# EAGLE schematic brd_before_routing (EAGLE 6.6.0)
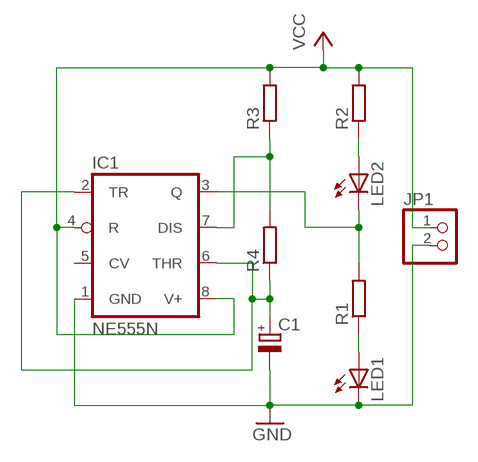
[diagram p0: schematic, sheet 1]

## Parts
C1  CPOL-EUE2.5-6  [E2,5-6]
IC1  NE555N  [DIL08]
JP1  PINHD-1X2  [1X02]
LED1  LED5MM  [LED5MM]
LED2  LED5MM  [LED5MM]
R1  R-EU_0207/10  [0207/10]
R2  R-EU_0207/10  [0207/10]
R3  R-EU_0207/10  [0207/10]
R4  R-EU_0207/10  [0207/10]

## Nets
GND: C1.- IC1.1(GND) JP1.2 LED1.K(C)
N$1: LED2.A R2.1
N$2: IC1.3(Q) LED2.K(C) R1.2
N$3: IC1.7(DIS) R3.1 R4.2
N$4: C1.+ IC1.2(TR) IC1.6(THR) R4.1
N$5: LED1.A R1.1
VCC: IC1.4(R) IC1.8(V+) JP1.1 R2.2 R3.2
Unconnected: IC1.5(CV)

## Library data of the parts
C1 = rcl:CPOL-EU: POLARIZED CAPACITOR, European symbol
IC1 = linear:*555: TIMER
JP1 = pinhead:PINHD-1X2: PIN HEADER
LED1 LED2 = led:LED: LED
R1-R4 = rcl:R-EU_: RESISTOR, European symbol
